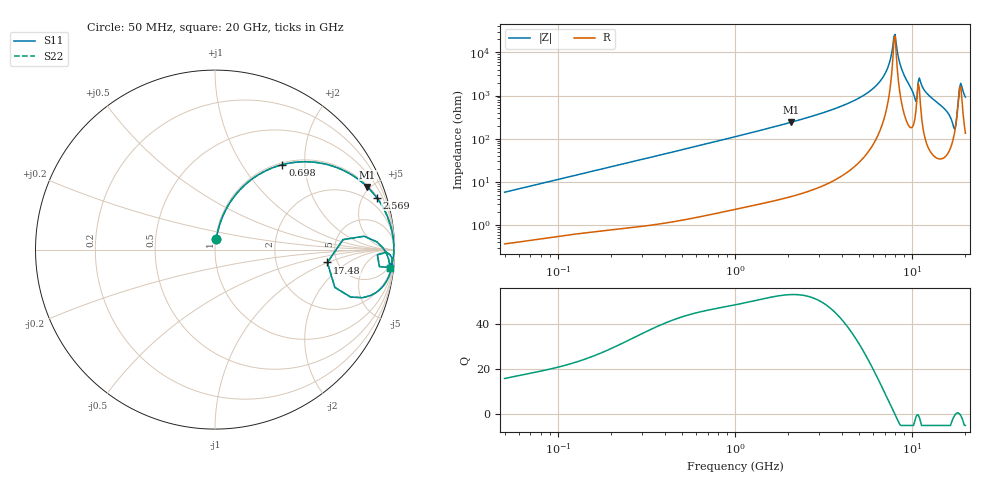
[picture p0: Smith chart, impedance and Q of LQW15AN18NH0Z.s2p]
!Murata Part Number: LQW15AN18NH0Z
!These Parameters are Measured in Series Mode Connection
!  o--[Z]--o
!Port1  Port2
!  o-------o
!Freq. Start=50[MHz] Stop=20[GHz], 401[Steps]
# Hz S RI R 50
!Freq.(Hz) S11(Real) S11(Imag) S21(Real) S21(Imag) S12(Real) S12(Imag) S22(Real) S22(Imag)
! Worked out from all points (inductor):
!   401 points, 50 MHz to 20 GHz, reference 50 ohm
!   read as one part in series: L = 18.1 nH near 51.52 MHz
!   highest Q = 52.8 at 2.083 GHz (marker M1), where L = 18.4 nH
!   self-resonance near 7.902 GHz
!   S11 on the Smith chart (normalised r, x): 50 MHz: 1.01, +0.11; 698 MHz: 1.03, +1.54; 2.569 GHz: 1.12, +6.17; 17.48 GHz: 4.16, -0.99; 20 GHz: 4, -18
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5e7  0.00686 0.0567  0.9931 -0.0567  0.9931 -0.0567  0.00686 0.0567
1.364002e8  0.0287 0.1474  0.9713 -0.1474  0.9713 -0.1474  0.0287 0.1474
3.721004e8  0.1509 0.3454  0.8491 -0.3454  0.8491 -0.3454  0.1509 0.3454
6.980337e8  0.3751 0.4734  0.6249 -0.4734  0.6249 -0.4734  0.3751 0.4734
1e9  0.5499 0.4872  0.4501 -0.4872  0.4501 -0.4872  0.5499 0.4872
2.083303e9  0.8488 0.3489  0.1512 -0.3489  0.1512 -0.3489  0.8488 0.3489
2.569357e9  0.9003 0.2901  0.0997 -0.2901  0.0997 -0.2901  0.9003 0.2901
2.728004e9  0.9124 0.2732  0.0876 -0.2732  0.0876 -0.2732  0.9124 0.2732
5.598765e9  0.9891 0.0854  0.0109 -0.0854  0.0109 -0.0854  0.9891 0.0854
6.701223e9  0.9948 0.0425  0.00521 -0.0425  0.00521 -0.0425  0.9948 0.0425
7.442007e9  0.9963 0.0172  0.00373 -0.0172  0.00373 -0.0172  0.9963 0.0172
7.784049e9  0.9965 0.0061  0.00353 -0.0061  0.00353 -0.0061  0.9965 0.0061
8.020766e9  0.9964 -0.00143  0.00357 0.00143  0.00357 0.00143  0.9964 -0.00143
8.774992e9  0.9954 -0.0253  0.00464 0.0253  0.00464 0.0253  0.9954 -0.0253
1.019291e10  0.9746 -0.0866  0.0254 0.0866  0.0254 0.0866  0.9746 -0.0866
1.115139e10  0.9843 -0.0445  0.0157 0.0445  0.0157 0.0445  0.9843 -0.0445
1.220001e10  0.986 -0.0899  0.014 0.0899  0.014 0.0899  0.986 -0.0899
1.646126e10  0.8663 -0.256  0.1337 0.256  0.1337 0.256  0.8663 -0.256
1.747767e10  0.6262 -0.0717  0.3738 0.0717  0.3738 0.0717  0.6262 -0.0717
1.800918e10  0.8306 0.0745  0.1694 -0.0745  0.1694 -0.0745  0.8306 0.0745
1.88369e10  0.9574 -0.0259  0.0426 0.0259  0.0426 0.0259  0.9574 -0.0259
2e10  0.9735 -0.1032  0.0265 0.1032  0.0265 0.1032  0.9735 -0.1032
